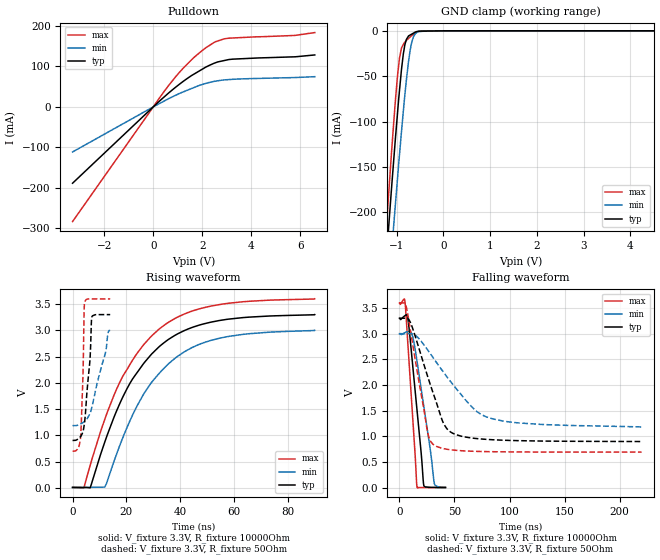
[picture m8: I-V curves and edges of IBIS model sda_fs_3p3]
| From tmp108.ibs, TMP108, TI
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|   sda_fs_3p3 Model
[Model]   sda_fs_3p3
Model_type   I/O_open_drain
Polarity   Non-Inverting
Vinl = 0.5
Vinh = 1.4
Vmeas = 1.65
Vref = 3.3
Cref = 2pF
Rref = 10000
|   typ   min   max
C_comp   6.770e-13   6.770e-13   7.186e-13
| Where nom  PVT is Nominal Process, 3.3V, 27C
|   Fast PVT is Strong Process,  3.6V, -40C
|   Slow PVT is Weak Process,   3V, 125C
[Voltage Range]   3.3   3   3.6
|Ambient Temperature   25   125   -40
|Junction Temperature
[Temperature Range]   27   125   -40
[Pullup Reference]   3.3   3   3.6
[Pulldown Reference]   0   0   0
[Power Clamp Reference]   3.3   3   3.6
[GND Clamp Reference]   0   0   0
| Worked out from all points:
|   slope of the pulldown table from 0 to 0.495 V, typ, clamps not added: 18.2 ohm
|   GND clamp passes 1 mA (typ) near -0.58 V on its own axis
|   falling waveform, V_fixture 3.3V, R_fixture 10000Ohm: 20-80 % time 8.9ns typ, 12.4ns min, 6.59ns max; typ from 3.3 V to 0.006 V
|   rising waveform, V_fixture 3.3V, R_fixture 10000Ohm: 20-80 % time 20.6ns typ, 20.4ns min, 20.9ns max; typ from 0.006 V to 3.3 V
|   falling waveform, V_fixture 3.3V, R_fixture 50Ohm: 20-80 % time 21.5ns typ, 40ns min, 13.7ns max; typ from 3.3 V to 0.901 V
|   rising waveform, V_fixture 3.3V, R_fixture 50Ohm: 20-80 % time 2.07ns typ, 5.22ns min, 897ps max; typ from 0.901 V to 3.3 V
[Pulldown]
|   Voltage   I(typ)   I(min)   I(max)
-3.3V     -188.7mA   -111.5mA   -283.5mA
633mV     34.54mA    20.43mA    53.27mA
1.246V    63.96mA    37.48mA    97.08mA
1.598V    78.58mA    46.12mA    118.4mA
2.012V    93.43mA    55.43mA    139.8mA
2.549V    109.1mA    63.56mA    161.1mA
2.934V    114.9mA    66.72mA    168.4mA
3.241V    117.9mA    67.98mA    170.2mA
5.774V    123.6mA    72.4mA     176.4mA
6.6V      128.3mA    74.58mA    183.5mA
[GND Clamp]
|   Voltage   I(typ)   I(min)   I(max)
-3.3V     -1.734A    -1.745A    -1.76A
-1.247V   -268.6mA   -335mA     -237mA
-1.119V   -179.7mA   -249.4mA   -140.5mA
-1.105V   -170.3mA   -240.6mA   -130.3mA
-1.037V   -124.9mA   -197.3mA   -82.91mA
-979.2mV  -88.9mA    -160.8mA   -48.16mA
-939.6mV  -65.66mA   -136.4mA   -30.04mA
-858mV    -25.6mA    -88.66mA   -15.11mA
-792mV    -9.495mA   -54.13mA   -10.6mA
-711mV    -4.601mA   -21.31mA   -6.699mA
-590.7mV  -1.091mA   -2.61mA    -2.149mA
6.6V      0A         0A         0A
[POWER Clamp]
|   Voltage   I(typ)   I(min)   I(max)
-3.3V     0A         0A         0A
-3.298V   0A         0A         0A
6.6V      0A         0A         0A
[Ramp]
R_load = 10000
|   typ   min   max
dV/dt_r   1.97654/2.05872e-08   1.79467/2.04269e-08   2.15758/2.08823e-08
dV/dt_f   1.97654/8.92016e-09   1.79467/1.24415e-08   2.15758/6.59614e-09
[Falling Waveform]
V_fixture = 3.3V
V_fixture_min = 3V
V_fixture_max = 3.6V
R_fixture = 10000Ohm
|   Time   V(typ)   V(min)   V(max)
0s        3.3V       3V         3.6V
4.39ns    3.341V     3.013V     3.678V
5.2ns     3.354V     3.022V     3.59V
7.16ns    3.346V     3.039V     2.969V
8.37ns    3.185V     3.044V     2.568V
11.58ns   2.487V     2.977V     1.515V
15.94ns   1.518V     2.469V     14.21mV
22.34ns   34.22mV    1.557V     5.651mV
31.79ns   8.352mV    76.63mV    4.683mV
41.81ns   6.413mV    11.94mV    4.222mV
[Rising Waveform]
V_fixture = 3.3V
V_fixture_min = 3V
V_fixture_max = 3.6V
R_fixture = 10000Ohm
|   Time   V(typ)   V(min)   V(max)
0s        5.762mV    8.86mV     4.03mV
4.28ns    4.16mV     7.699mV    9.796mV
6.52ns    -1.937mV   8.196mV    421.2mV
12ns      873.9mV    12.11mV    1.307V
21.37ns   1.993V     1.28V      2.352V
26.73ns   2.388V     1.809V     2.744V
33.07ns   2.726V     2.228V     3.059V
41.41ns   2.992V     2.585V     3.308V
51.52ns   3.157V     2.809V     3.463V
90.09ns   3.3V       3V         3.6V
[Falling Waveform]
V_fixture = 3.3V
V_fixture_min = 3V
V_fixture_max = 3.6V
R_fixture = 50Ohm
|   Time   V(typ)   V(min)   V(max)
0s        3.3V       3V         3.6V
6.38ns    3.301V     3.001V     3.508V
11.6ns    3.129V     2.996V     2.855V
25.75ns   2.16V      2.68V      1.066V
32.95ns   1.7V       2.461V     812.5mV
39.34ns   1.289V     2.271V     766.9mV
46.1ns    1.092V     2.078V     741.8mV
70.17ns   959mV      1.486V     709.6mV
83.27ns   937.7mV    1.352V     703.7mV
220ns     901.2mV    1.184V     695.2mV
[Rising Waveform]
V_fixture = 3.3V
V_fixture_min = 3V
V_fixture_max = 3.6V
R_fixture = 50Ohm
|   Time   V(typ)   V(min)   V(max)
0s        901.2mV    1.184V     695.2mV
3ns       976.4mV    1.215V     956.9mV
3.78ns    1.054V     1.238V     1.983V
3.98ns    1.088V     1.245V     2.381V
4.27ns    1.175V     1.256V     3.309V
4.48ns    1.254V     1.265V     3.527V
6.47ns    2.43V      1.413V     3.6V
7.2ns     3.26V      1.537V     3.6V
13.29ns   3.3V       2.972V     3.6V
14ns      3.3V       3V         3.6V
